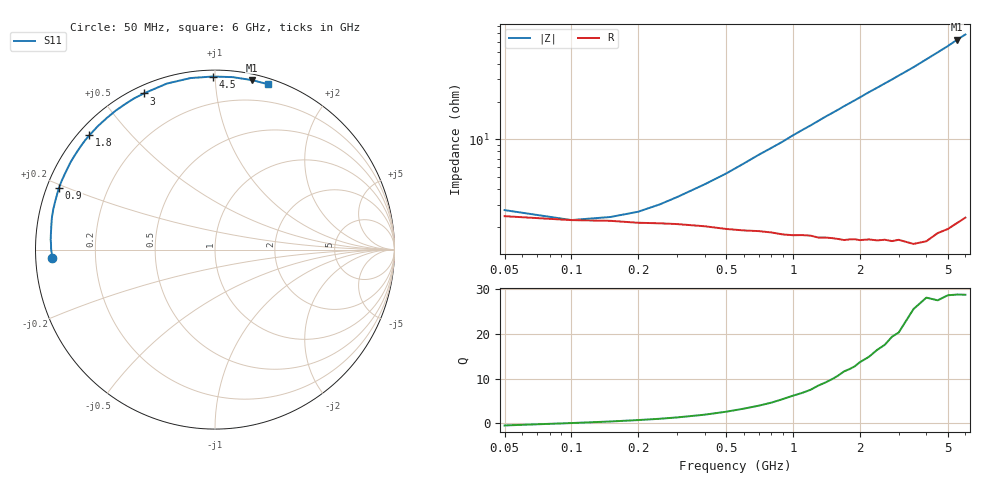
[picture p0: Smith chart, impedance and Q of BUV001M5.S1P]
! Infineon Technologies  Discrete & RF Semiconductors
! BB 833
! Si Tuning Diode in SOD323
! VR =
! S-Parameters:  June  1999
# GHz  S  MA  R  50
!  f  S11
! GHz  MAG  ANG
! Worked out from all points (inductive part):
!   34 points, 50 MHz to 6 GHz, reference 50 ohm
!   read as one part to ground: L = 1.66 nH near 600 MHz
!   highest Q = 28.8 at 5.5 GHz (marker M1), where L = 1.8 nH
!   S11 on the Smith chart (normalised r, x): 50 MHz: 0.05, -0.02; 900 MHz: 0.03, +0.19; 1.8 GHz: 0.03, +0.39; 3 GHz: 0.03, +0.64; 4.5 GHz: 0.04, +0.99; 6 GHz: 0.05, +1.37
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0.05  0.907 -177.2
0.1  0.9131 179.8
0.15  0.9142 178.0
0.2  0.9171 176.5
0.3  0.9192 173.7
0.5  0.9264 168.6
0.6  0.9286 166.0
0.7  0.9299 163.4
0.8  0.9319 161.0
0.9  0.9348 158.6
1  0.9362 156.0
1.3  0.9406 148.9
1.4  0.9413 146.5
1.6  0.9441 142.1
1.7  0.9459 139.8
1.8  0.946 137.7
2  0.9483 133.5
2.2  0.9493 129.3
2.4  0.9517 125.5
2.6  0.9528 121.7
2.8  0.9555 118.1
3  0.9562 114.5
3.5  0.9632 106.2
4  0.9654 98.1
4.5  0.9643 90.8
5  0.9659 84.2
5.5  0.9667 77.7
6  0.9675 72.3
